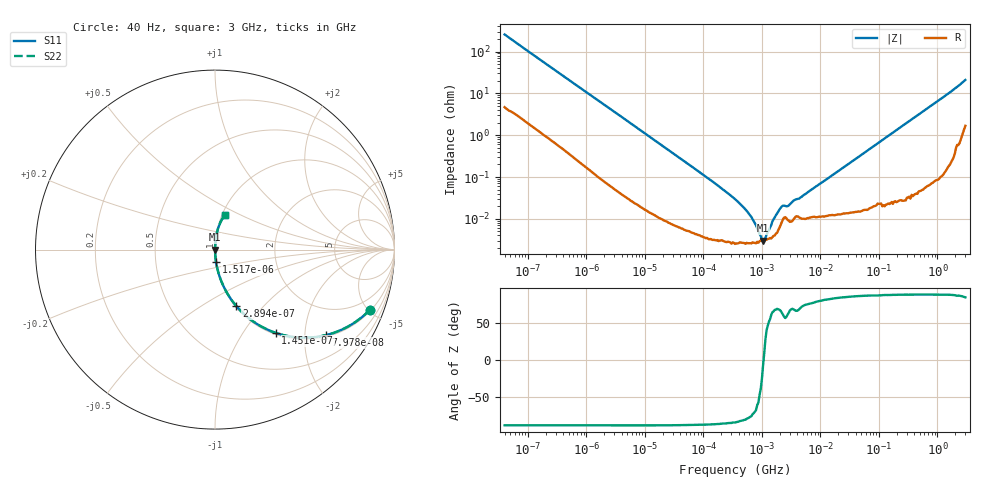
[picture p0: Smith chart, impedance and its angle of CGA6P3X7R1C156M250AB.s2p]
! S-parameter Generated by TDK Corporation
! Copyright(C) 2015 TDK Corporation.
! All Rights Reserved.
! TDK P/N: CGA6P3X7R1C156M250AB (Multilayer Ceramic Chip Capacitors)
! Property: C=15uF
! Size(LxWxT): 3.2x2.5x2.5mm, 0.126x0.098x0.098inches
! Model Type: s2p (Touchstone File Format Version 1.0)
! Frequency: DC=Yes Start=0.00004MHz Stop=3000MHz 396points Log-sweep
! Note: This model was converted from impedance.
! Model Generated on Jun. 23, 2015
! Hash(MD5):
! Port Assignments:
!  1 ---| |--- 2
! Applicable Conditions:
!  Temperature = 25 degC
!  DC Bias Voltage = 0 V
!  Small Signal Operation
! Terms and conditions regarding TDK Simulation Models
! (1)This simulation model is being provided solely for informational purposes. Please refer to the specifications of the products in terms of detailed characteristics of such products.
! (2)In no event shall TDK Corporation of any of its subsidiaries be liable for any loss or damage arising, directly or indirectly,
!  From any information contained in this simulation model, including, but not limited to loss or damages arising from any inaccuracies, omissions or errors in connection with such information.
! (3)Any and all copyrights on this simulation model are owned by TDK Corporation.
!  Duplication or redistribution of this simulation model without prior written permission from TDK Corporation is prohibited.
! (4)This simulation model is subject to any modification or change without any prior notice.
! (5)Neither TDK Corporation nor any of its subsidiaries shall make any warranty, express or implied,
!  Including but not limited to the correctness, implied warranties of merchantability and fitness for a particular purpose with respect to this simulation models.
! (6)The use of this simulation model shall be deemed to have consented to the terms and conditions hereof.
# MHz S MA R 50
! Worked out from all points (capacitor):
!   395 points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, 40 Hz to 3 GHz, reference 50 ohm
!   read as one part in series: C = 15.6 uF near 41.88 Hz
!   lowest |Z| = 2.98 mohm at 1.045 MHz (marker M1)
!   series resonance near 1.066 MHz, so ESL is about 1.4 nH
!   S11 on the Smith chart (normalised r, x): 40 Hz: 1.09, -5.13; 79.78 Hz: 1.05, -2.57; 145.1 Hz: 1.03, -1.42; 289.4 Hz: 1.01, -0.72; 1.517 kHz: 1.00, -0.14; 3 GHz: 1.03, +0.42
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4e-05  0.9259 -21.2  0.3612 67.8  0.3612 67.8  0.9259 -21.2
7.977595e-05  0.7816 -37.5  0.6092 51.4  0.6092 51.4  0.7816 -37.5
0.0001451139  0.574 -53.9  0.8082 35.0  0.8082 35.0  0.574 -53.9
0.000289415  0.3367 -69.3  0.9356 19.7  0.9356 19.7  0.3367 -69.3
0.000834128  0.1264 -81.8  0.99 7.3  0.99 7.3  0.1264 -81.8
0.001517294  0.07078 -85.1  0.9965 4.1  0.9965 4.1  0.07078 -85.1
0.01739424  0.006384 -88.7  0.9999 0.4  0.9999 0.4  0.006384 -88.7
0.1512921  0.0007373 -87.5  1 0.0  1 0.0  0.0007373 -87.5
0.3464102  0.0002953 -85.1  1 0.0  1 0.0  0.0002953 -85.1
0.5241768  0.0001675 -81.3  1 0.0  1 0.0  0.0001675 -81.3
0.69088  9.859e-05 -73.9  1 0.0  1 0.0  9.859e-05 -73.9
1.045418  2.98e-05 -7.3  1 0.0  1 0.0  2.98e-05 -7.3
1.581893  9.699e-05 66.3  1 -0.0  1 -0.0  9.699e-05 66.3
2.084979  0.0001826 67.1  0.9999 -0.0  0.9999 -0.0  0.0001826 67.1
2.286002  0.0002067 61.9  0.9999 -0.0  0.9999 -0.0  0.0002067 61.9
2.748062  0.0002007 62.0  0.9999 -0.0  0.9999 -0.0  0.0002007 62.0
3.459106  0.0002721 69.1  0.9999 -0.0  0.9999 -0.0  0.0002721 69.1
4.354128  0.0003073 69.5  0.9999 -0.0  0.9999 -0.0  0.0003073 69.5
7.22376  0.0005132 77.6  0.9999 -0.0  0.9999 -0.0  0.0005132 77.6
150.6385  0.01002 88.1  0.9997 -0.6  0.9997 -0.6  0.01002 88.1
994.0817  0.06429 85.6  0.9971 -3.7  0.9971 -3.7  0.06429 85.6
3000  0.2021 73.8  0.9633 -11.6  0.9633 -11.6  0.2021 73.8
